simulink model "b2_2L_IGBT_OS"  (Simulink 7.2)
settings: Solver=ode3  SolverMode=SingleTasking  StartTime=0.0  StopTime=0.1  FixedStep=10e-6  MaxStep=1e-5  RelTol=1e-4  AbsTol=1e-4

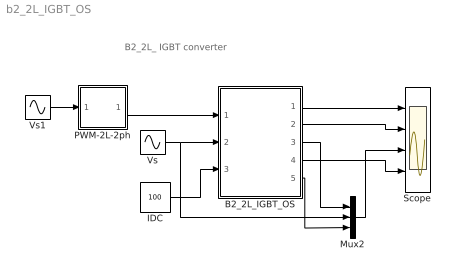
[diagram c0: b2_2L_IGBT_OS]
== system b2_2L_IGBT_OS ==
  note: B2_2L_ IGBT converter
  B2_2L_IGBT_OS : Subsystem  mask(B2-2-Level IGBT Converter){LS=2e-3, C=10e-3, VC0=400, RL=10e5}
      mask prompts: LS "Source Inductance"; C "Load Cap"; VC0 "Initial Cap Voltage"; RL "Load Resistance"
      mask help: Input Vector u: u[0]= IGBT1.gate u[1]= IGBT2.gate u[2]= IGBT3.gate u[3]= IGBT4.gate u[4]= V1.V u[5]= IDC.i Output Vector y: y[0]= T1.I y[1]= D1.I y[2]= T1.V y[3]= T2.I y[4]= D2.I y[5]= T2.V y[6]= LS1.I y[7]= DC.V y[8]= Va.V Parameter Vector p: p[0]= Ls.L p[1]= C1.C p[2]= C1.vC0 p[3]= R1.r You can pause the simulation during running, change the Parameters you want and continue the Simulation
  IDC : Constant  Value=100
  Mux2 : Mux  Inputs=3
  PWM-2L-2ph : Subsystem  mask(PWM-2L-2PH){FT=900, PHT=0, DT=1e-6}
      mask prompts: FT "Triangular Frequency"; PHT "Trian. Phase Angle (Degree)"; DT "Dead Time"
      mask help: Pulse Width Modulation for 2 Legs of 2-Level Converter
  Scope : Scope  NumInputPorts=4
  Vs : Sin  Amplitude=230*sqrt(2)  Frequency=50*2*pi  SampleTime=0
  Vs1 : Sin  Amplitude=0.74  Frequency=50*2*pi  Phase=-pi/6  SampleTime=0
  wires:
  IDC/1 -> B2_2L_IGBT_OS/3(iDC)
  B2_2L_IGBT_OS/1(iT1,iD1,vT1) -> Scope/1
  B2_2L_IGBT_OS/2(iT2,iD2,vT2) -> Scope/2
  B2_2L_IGBT_OS/4(vDC) -> Scope/4
  Vs/1 -> B2_2L_IGBT_OS/2(vS), Mux2/2
  Vs1/1 -> PWM-2L-2ph/1(I1)
  B2_2L_IGBT_OS/3(iLs) -> Mux2/1
  Mux2/1 -> Scope/3
  B2_2L_IGBT_OS/5(va) -> Mux2/3
  PWM-2L-2ph/1(O1) -> B2_2L_IGBT_OS/1(SWs)

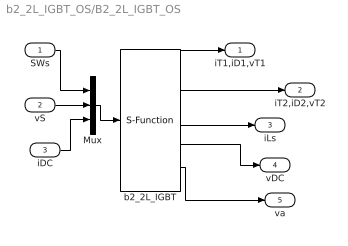
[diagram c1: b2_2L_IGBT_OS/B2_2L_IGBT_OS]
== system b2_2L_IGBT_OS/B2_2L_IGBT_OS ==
  SWs : Inport  OutDataType=sfix(16)  OutScaling=2^0
  vS : Inport  Port=2  OutDataType=sfix(16)  OutScaling=2^0
  iDC : Inport  Port=3  OutDataType=sfix(16)  OutScaling=2^0
  Mux : Mux  Inputs="[4  1  1]"
  b2_2L_IGBT : S-Function  FunctionName=s_b2_2L_IGBT_OS  Parameters="[ LS  C  VC0 RL]"  EnableBusSupport=off
  iT1,iD1,vT1 : Outport  OutDataType=sfix(16)  OutScaling=2^0
  iT2,iD2,vT2 : Outport  Port=2  OutDataType=sfix(16)  OutScaling=2^0
  iLs : Outport  Port=3  OutDataType=sfix(16)  OutScaling=2^0
  vDC : Outport  Port=4  OutDataType=sfix(16)  OutScaling=2^0
  va : Outport  Port=5  OutDataType=sfix(16)  OutScaling=2^0
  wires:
  b2_2L_IGBT/5 -> va/1
  SWs/1 -> Mux/1
  vS/1 -> Mux/2
  b2_2L_IGBT/1 -> iT1,iD1,vT1/1
  b2_2L_IGBT/2 -> iT2,iD2,vT2/1
  b2_2L_IGBT/3 -> iLs/1
  iDC/1 -> Mux/3
  Mux/1 -> b2_2L_IGBT/1
  b2_2L_IGBT/4 -> vDC/1

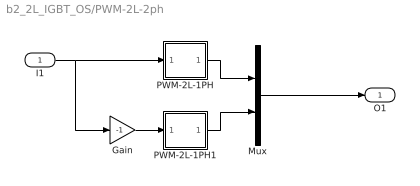
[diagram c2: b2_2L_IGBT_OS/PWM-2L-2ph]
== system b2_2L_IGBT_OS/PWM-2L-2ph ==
  I1 : Inport  OutDataType=sfix(16)  OutScaling=2^0
  Gain : Gain  Gain=-1  ParameterDataType=sfix(16)  ParameterScaling=2^0  OutDataType=sfix(16)  OutScaling=2^0
  Mux : Mux  Inputs=2
  PWM-2L-1PH : Subsystem  mask(PWM-2L-1PH){FT=FT, PHT=PHT, DT=DT}
      mask prompts: FT "Triangular Frequency"; PHT "Trian. Phase Angle (Degree)"; DT "Dead Time"
      mask help: Pulse Width Modulation for 1 Phase Converter
  PWM-2L-1PH1 : Subsystem  mask(PWM-2L-1PH){FT=FT, PHT=PHT, DT=DT}
      mask prompts: FT "Triangular Frequency"; PHT "Trian. Phase Angle (Degree)"; DT "Dead Time"
      mask help: Pulse Width Modulation for 1 Phase Converter
  O1 : Outport
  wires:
  Gain/1 -> PWM-2L-1PH1/1(In1)
  I1/1 -> Gain/1, PWM-2L-1PH/1(In1)
  PWM-2L-1PH/1(Out1) -> Mux/1
  PWM-2L-1PH1/1(Out1) -> Mux/2
  Mux/1 -> O1/1

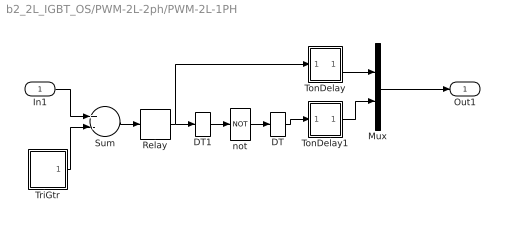
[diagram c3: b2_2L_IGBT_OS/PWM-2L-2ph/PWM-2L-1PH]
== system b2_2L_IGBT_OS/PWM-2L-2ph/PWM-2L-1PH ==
  In1 : Inport  OutDataType=sfix(16)  OutScaling=2^0
  DT : DataTypeConversion
  DT1 : DataTypeConversion
  Mux : Mux  Inputs=2
  Relay : Relay  OutDataType=sfix(16)  OutScaling=2^0
  Sum : Sum  Inputs=+-  OutDataType=sfix(16)  OutScaling=2^0
  TonDelay : Subsystem  mask(TonDelay){DT=DT}
      mask prompts: DT "Dead Time"
      mask help: Turn on dead time to protect against short circuit of the converter leg
  TonDelay1 : Subsystem  mask(TonDelay){DT=DT}
      mask prompts: DT "Dead Time"
      mask help: Turn on dead time to protect against short circuit of the converter leg
  TriGtr : Subsystem  mask(TriGtr){T=1/FT, Td=PHT/FT/360}
      mask prompts: T "Period Time"; Td "Time Delay"
      mask help: Triangular Wave Generator with variable time delay
  not : Logic  Operator=NOT  Inputs=1
  Out1 : Outport  InitialOutput=0
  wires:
  DT1/1 -> not/1
  DT/1 -> TonDelay1/1(s1)
  In1/1 -> Sum/1
  TriGtr/1(O) -> Sum/2
  Sum/1 -> Relay/1
  not/1 -> DT/1
  TonDelay1/1(s1d) -> Mux/2
  Relay/1 -> DT1/1, TonDelay/1(s1)
  TonDelay/1(s1d) -> Mux/1
  Mux/1 -> Out1/1

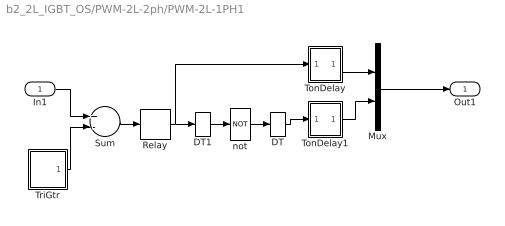
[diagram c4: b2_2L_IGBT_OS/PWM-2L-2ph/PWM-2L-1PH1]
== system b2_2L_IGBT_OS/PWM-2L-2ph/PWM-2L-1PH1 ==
  In1 : Inport  OutDataType=sfix(16)  OutScaling=2^0
  DT : DataTypeConversion
  DT1 : DataTypeConversion
  Mux : Mux  Inputs=2
  Relay : Relay  OutDataType=sfix(16)  OutScaling=2^0
  Sum : Sum  Inputs=+-  OutDataType=sfix(16)  OutScaling=2^0
  TonDelay : Subsystem  mask(TonDelay){DT=DT}
      mask prompts: DT "Dead Time"
      mask help: Turn on dead time to protect against short circuit of the converter leg
  TonDelay1 : Subsystem  mask(TonDelay){DT=DT}
      mask prompts: DT "Dead Time"
      mask help: Turn on dead time to protect against short circuit of the converter leg
  TriGtr : Subsystem  mask(TriGtr){T=1/FT, Td=PHT/FT/360}
      mask prompts: T "Period Time"; Td "Time Delay"
      mask help: Triangular Wave Generator with variable time delay
  not : Logic  Operator=NOT  Inputs=1
  Out1 : Outport  InitialOutput=0
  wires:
  Mux/1 -> Out1/1
  TonDelay/1(s1d) -> Mux/1
  Relay/1 -> TonDelay/1(s1), DT1/1
  TonDelay1/1(s1d) -> Mux/2
  not/1 -> DT/1
  Sum/1 -> Relay/1
  TriGtr/1(O) -> Sum/2
  In1/1 -> Sum/1
  DT/1 -> TonDelay1/1(s1)
  DT1/1 -> not/1

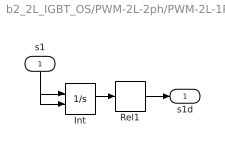
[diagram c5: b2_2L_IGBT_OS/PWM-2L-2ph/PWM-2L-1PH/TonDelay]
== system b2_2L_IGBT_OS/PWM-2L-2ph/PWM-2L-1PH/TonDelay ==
  s1 : Inport  Orientation=down  OutDataType=sfix(16)  OutScaling=2^0
  Int : Integrator  ExternalReset=falling
  Rel1 : Relay  OnSwitchValue=DT  OutDataType=sfix(16)  OutScaling=2^0
  s1d : Outport  InitialOutput=0
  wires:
  Int/1 -> Rel1/1
  s1/1 -> Int/2, Int/1
  Rel1/1 -> s1d/1

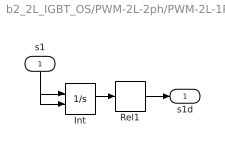
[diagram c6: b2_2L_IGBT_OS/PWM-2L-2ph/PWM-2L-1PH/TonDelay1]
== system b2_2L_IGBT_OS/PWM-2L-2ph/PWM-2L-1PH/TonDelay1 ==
  s1 : Inport  Orientation=down  OutDataType=sfix(16)  OutScaling=2^0
  Int : Integrator  ExternalReset=falling
  Rel1 : Relay  OnSwitchValue=DT  OutDataType=sfix(16)  OutScaling=2^0
  s1d : Outport  InitialOutput=0
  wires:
  Int/1 -> Rel1/1
  s1/1 -> Int/2, Int/1
  Rel1/1 -> s1d/1

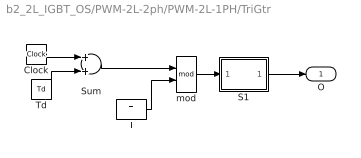
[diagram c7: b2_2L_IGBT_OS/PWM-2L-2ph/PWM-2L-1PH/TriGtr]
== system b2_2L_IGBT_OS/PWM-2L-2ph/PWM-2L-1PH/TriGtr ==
  Clock : Clock
  S1 : Subsystem
  Sum : Sum  OutDataType=sfix(16)  OutScaling=2^0
  T : Constant  Value=T  OutDataType=sfix(16)  OutScaling=2^0
  Td : Constant  Value=Td  OutDataType=sfix(16)  OutScaling=2^0
  mod : Math  Operator=mod
  O : Outport  InitialOutput=0
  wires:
  mod/1 -> S1/1(I1)
  S1/1(O1) -> O/1
  Clock/1 -> Sum/1
  T/1 -> mod/2
  Sum/1 -> mod/1
  Td/1 -> Sum/2

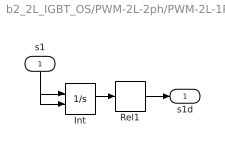
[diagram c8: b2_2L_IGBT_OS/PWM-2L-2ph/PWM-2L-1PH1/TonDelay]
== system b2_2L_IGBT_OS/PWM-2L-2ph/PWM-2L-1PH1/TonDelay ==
  s1 : Inport  Orientation=down  OutDataType=sfix(16)  OutScaling=2^0
  Int : Integrator  ExternalReset=falling
  Rel1 : Relay  OnSwitchValue=DT  OutDataType=sfix(16)  OutScaling=2^0
  s1d : Outport  InitialOutput=0
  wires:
  Rel1/1 -> s1d/1
  s1/1 -> Int/1, Int/2
  Int/1 -> Rel1/1

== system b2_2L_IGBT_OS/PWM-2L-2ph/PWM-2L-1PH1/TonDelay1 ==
  s1 : Inport  Orientation=down  OutDataType=sfix(16)  OutScaling=2^0
  Int : Integrator  ExternalReset=falling
  Rel1 : Relay  OnSwitchValue=DT  OutDataType=sfix(16)  OutScaling=2^0
  s1d : Outport  InitialOutput=0
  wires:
  Rel1/1 -> s1d/1
  s1/1 -> Int/1, Int/2
  Int/1 -> Rel1/1

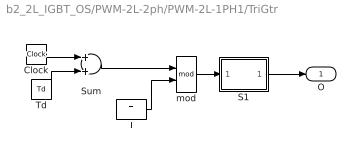
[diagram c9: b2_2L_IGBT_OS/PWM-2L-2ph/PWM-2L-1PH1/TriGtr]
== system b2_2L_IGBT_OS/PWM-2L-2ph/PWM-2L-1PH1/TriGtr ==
  Clock : Clock
  S1 : Subsystem
  Sum : Sum  OutDataType=sfix(16)  OutScaling=2^0
  T : Constant  Value=T  OutDataType=sfix(16)  OutScaling=2^0
  Td : Constant  Value=Td  OutDataType=sfix(16)  OutScaling=2^0
  mod : Math  Operator=mod
  O : Outport  InitialOutput=0
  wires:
  Td/1 -> Sum/2
  Sum/1 -> mod/1
  T/1 -> mod/2
  Clock/1 -> Sum/1
  S1/1(O1) -> O/1
  mod/1 -> S1/1(I1)

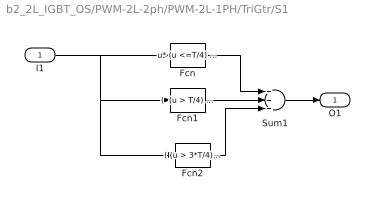
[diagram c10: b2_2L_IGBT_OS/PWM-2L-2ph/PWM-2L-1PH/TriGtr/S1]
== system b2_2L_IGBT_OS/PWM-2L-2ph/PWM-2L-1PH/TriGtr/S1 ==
  I1 : Inport  OutDataType=sfix(16)  OutScaling=2^0
  Fcn : Fcn  Expr=u* (u <=T/4) * 4/T
  Fcn1 : Fcn  Expr="(  (u > T/4) && ( u <=3*T/4) )* ( 1 - (u-T/4) *4/T )"
  Fcn2 : Fcn  Expr=( (u > 3*T/4)&& (u<=T)) * ( ((u -3*T/4)* 4/T )-1 )
  Sum1 : Sum  Inputs=+++  OutDataType=sfix(16)  OutScaling=2^0
  O1 : Outport
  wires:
  Fcn2/1 -> Sum1/3
  Fcn1/1 -> Sum1/2
  Fcn/1 -> Sum1/1
  Sum1/1 -> O1/1
  I1/1 -> Fcn/1, Fcn2/1, Fcn1/1

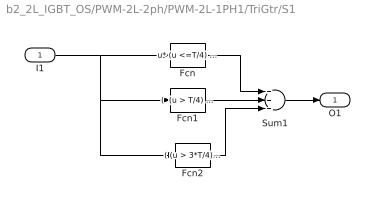
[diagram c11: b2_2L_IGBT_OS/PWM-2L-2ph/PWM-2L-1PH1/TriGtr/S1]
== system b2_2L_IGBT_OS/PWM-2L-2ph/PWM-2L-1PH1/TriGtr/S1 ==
  I1 : Inport  OutDataType=sfix(16)  OutScaling=2^0
  Fcn : Fcn  Expr=u* (u <=T/4) * 4/T
  Fcn1 : Fcn  Expr="(  (u > T/4) && ( u <=3*T/4) )* ( 1 - (u-T/4) *4/T )"
  Fcn2 : Fcn  Expr=( (u > 3*T/4)&& (u<=T)) * ( ((u -3*T/4)* 4/T )-1 )
  Sum1 : Sum  Inputs=+++  OutDataType=sfix(16)  OutScaling=2^0
  O1 : Outport
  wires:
  I1/1 -> Fcn1/1, Fcn2/1, Fcn/1
  Sum1/1 -> O1/1
  Fcn/1 -> Sum1/1
  Fcn1/1 -> Sum1/2
  Fcn2/1 -> Sum1/3
